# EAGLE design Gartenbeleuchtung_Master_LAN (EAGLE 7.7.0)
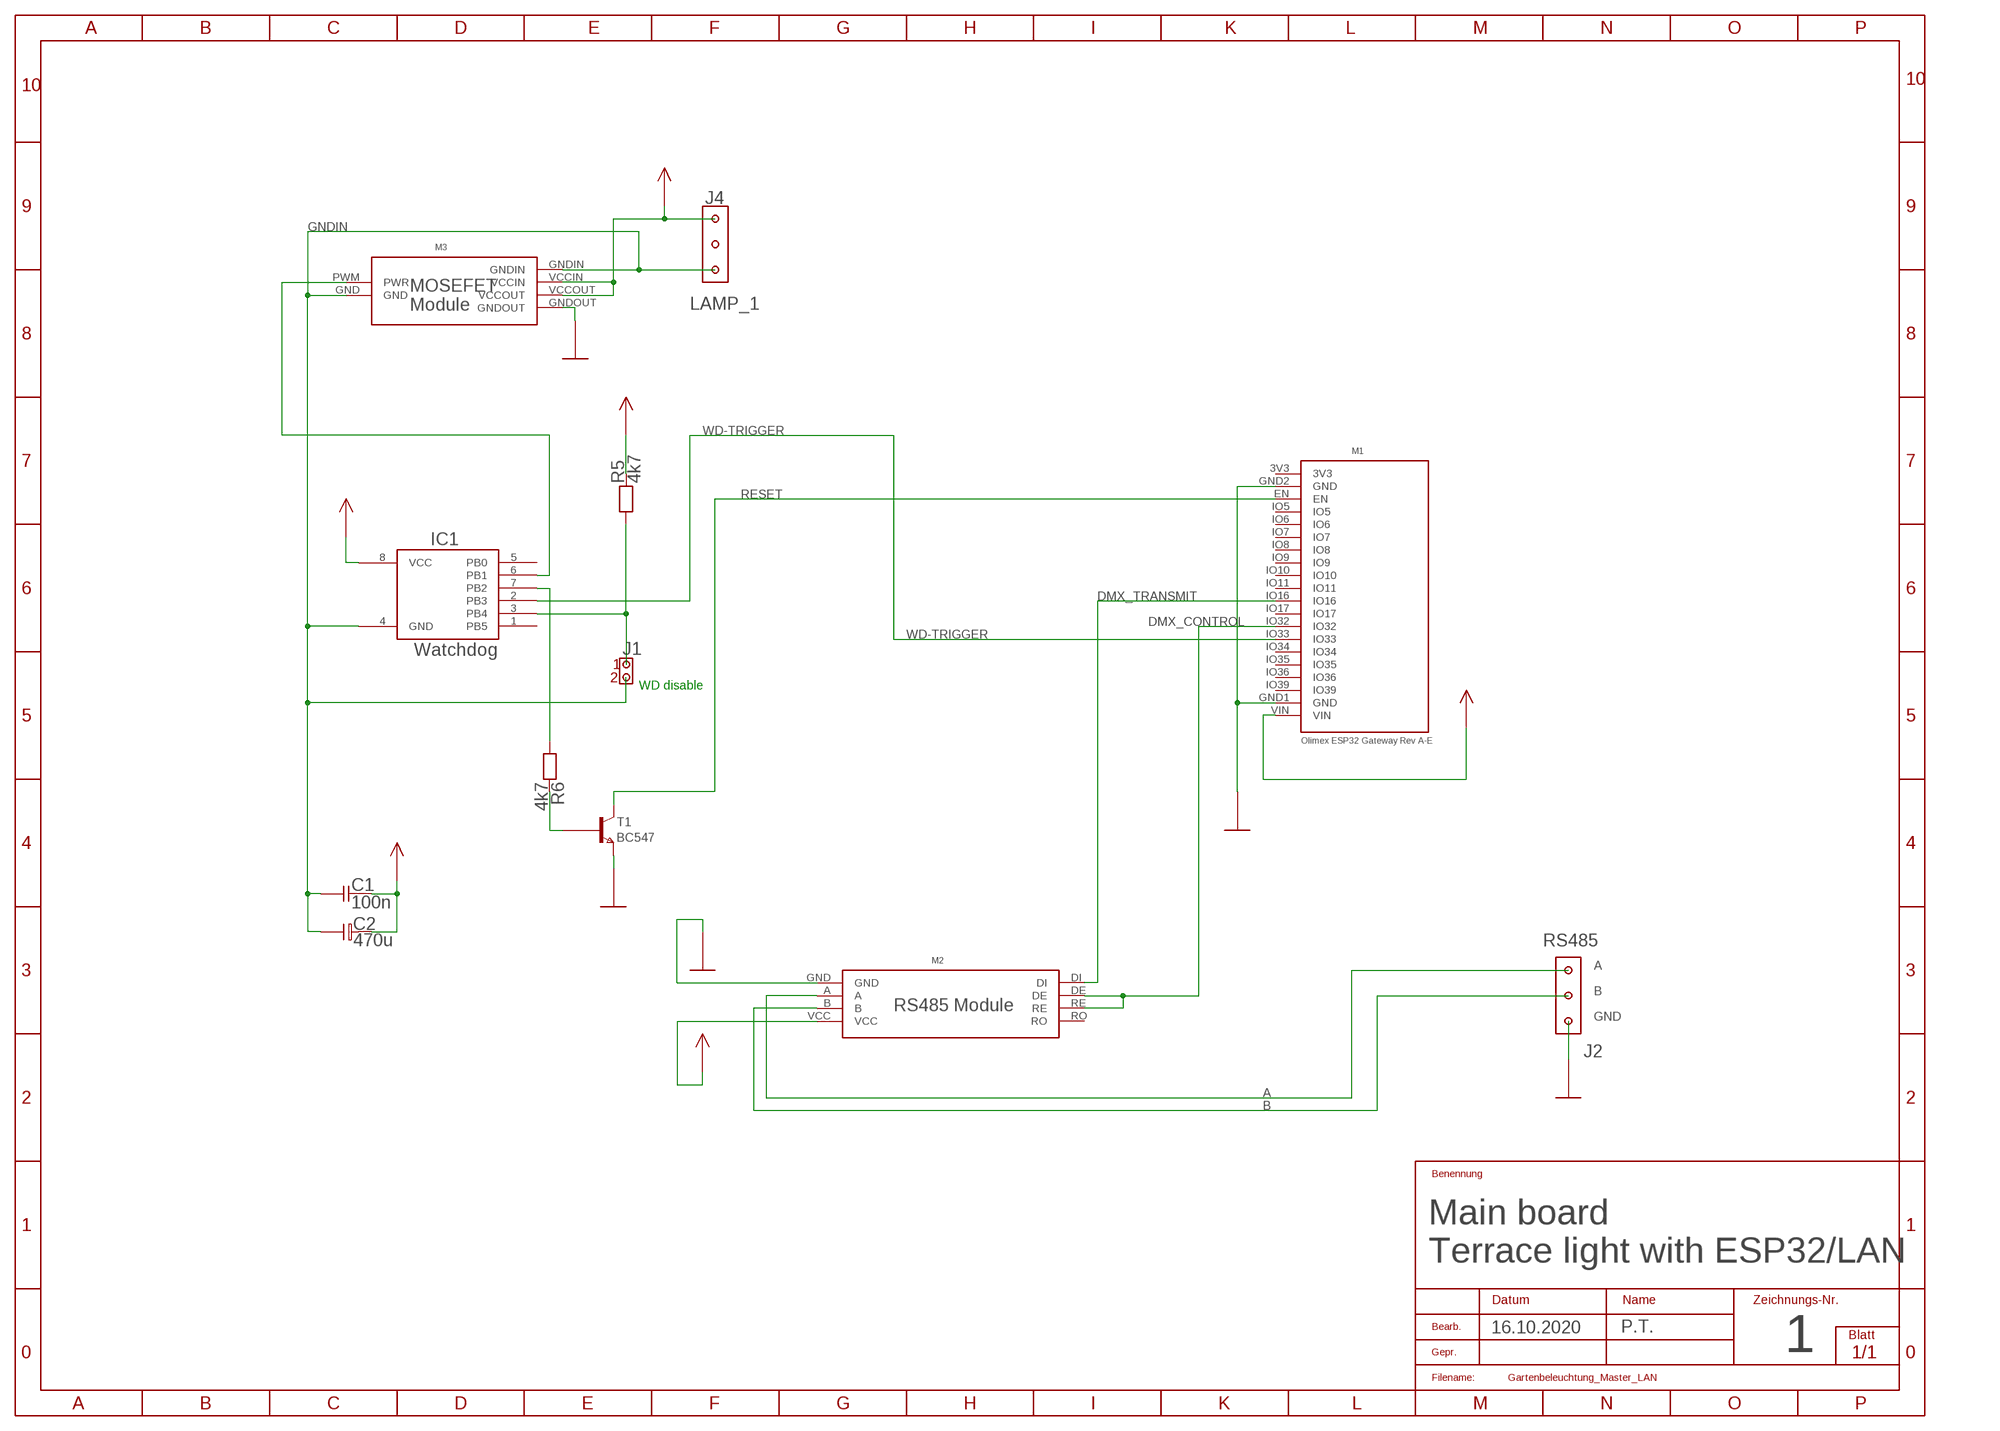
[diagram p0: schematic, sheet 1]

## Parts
C1  100n  CAP02  [CAP02B]
C2  470u  ELK02LI  [ELKOL02B]
IC1  Watchdog  ATINY13A  [DIL8]
J1  WD disable  CON02X1  [CON02X1]
J2  RS485  POWER3X1  [POWER3X1]
J4  LAMP_1  POWER3X1  [POWER3X1]
M1  ESP32-GATEWAY-E  [ESP32-GATEWAY-E]
M2  RS485  [RS485]
M3  MOSFET  [MOSFET]
R5  4k7  RES04  [RES04B]
R6  4k7  RES04  [RES04B]
T1  BC547  BC237  [TO92A]

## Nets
A: J2.3 M2.A
B: J2.2 M2.B
DMX_CONTROL: M1.IO32 M2.DE M2.RE
DMX_TRANSMIT: M1.IO16 M2.DI
GND: J2.1 M1.GND1(GND) M1.GND2(GND) M2.GND M3.GNDOUT T1.3(E)
GNDIN: C1.1 C2.N IC1.4(GND) J1.2 J4.1 M3.GND M3.GNDIN
N$4: IC1.3(PB4) J1.1 R5.1
N$7: IC1.7(PB2) R6.1
N$8: IC1.6(PB1) M3.PWM(PWR)
N$9: R6.2 T1.2(B)
RESET: M1.EN T1.1(C)
VCC: C1.2 C2.P IC1.8(VCC) J4.3 M1.VIN M2.VCC M3.VCCIN M3.VCCOUT R5.2
WD-TRIGGER: IC1.2(PB3) M1.IO33
Unconnected: IC1.1(PB5) IC1.5(PB0) J4.2 M1.IO5 M1.IO6 M1.IO7 M1.IO8 M1.IO9 M1.IO10 M1.IO11 M1.IO17 M1.IO34 M1.IO35 M1.IO36 M1.IO39 M2.RO

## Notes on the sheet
- WD disable
- Main board
- Terrace light with ESP32/LAN
- 16.10.2020 | P.T.
- 1

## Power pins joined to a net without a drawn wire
3V3: M1.3V3

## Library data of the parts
C1 = Discrete:CAP02
C2 = Discrete:ELK02LI
IC1 = Processor:ATINY13A
J1 = Connector 1:CON02X1
J2 J4 = Connector 2:POWER3X1
M1 = Giess:ESP32-GATEWAY-E
M2 = Giess:RS485
M3 = Giess:MOSFET
R5 R6 = Discrete:RES04
T1 = Transistor:BC237

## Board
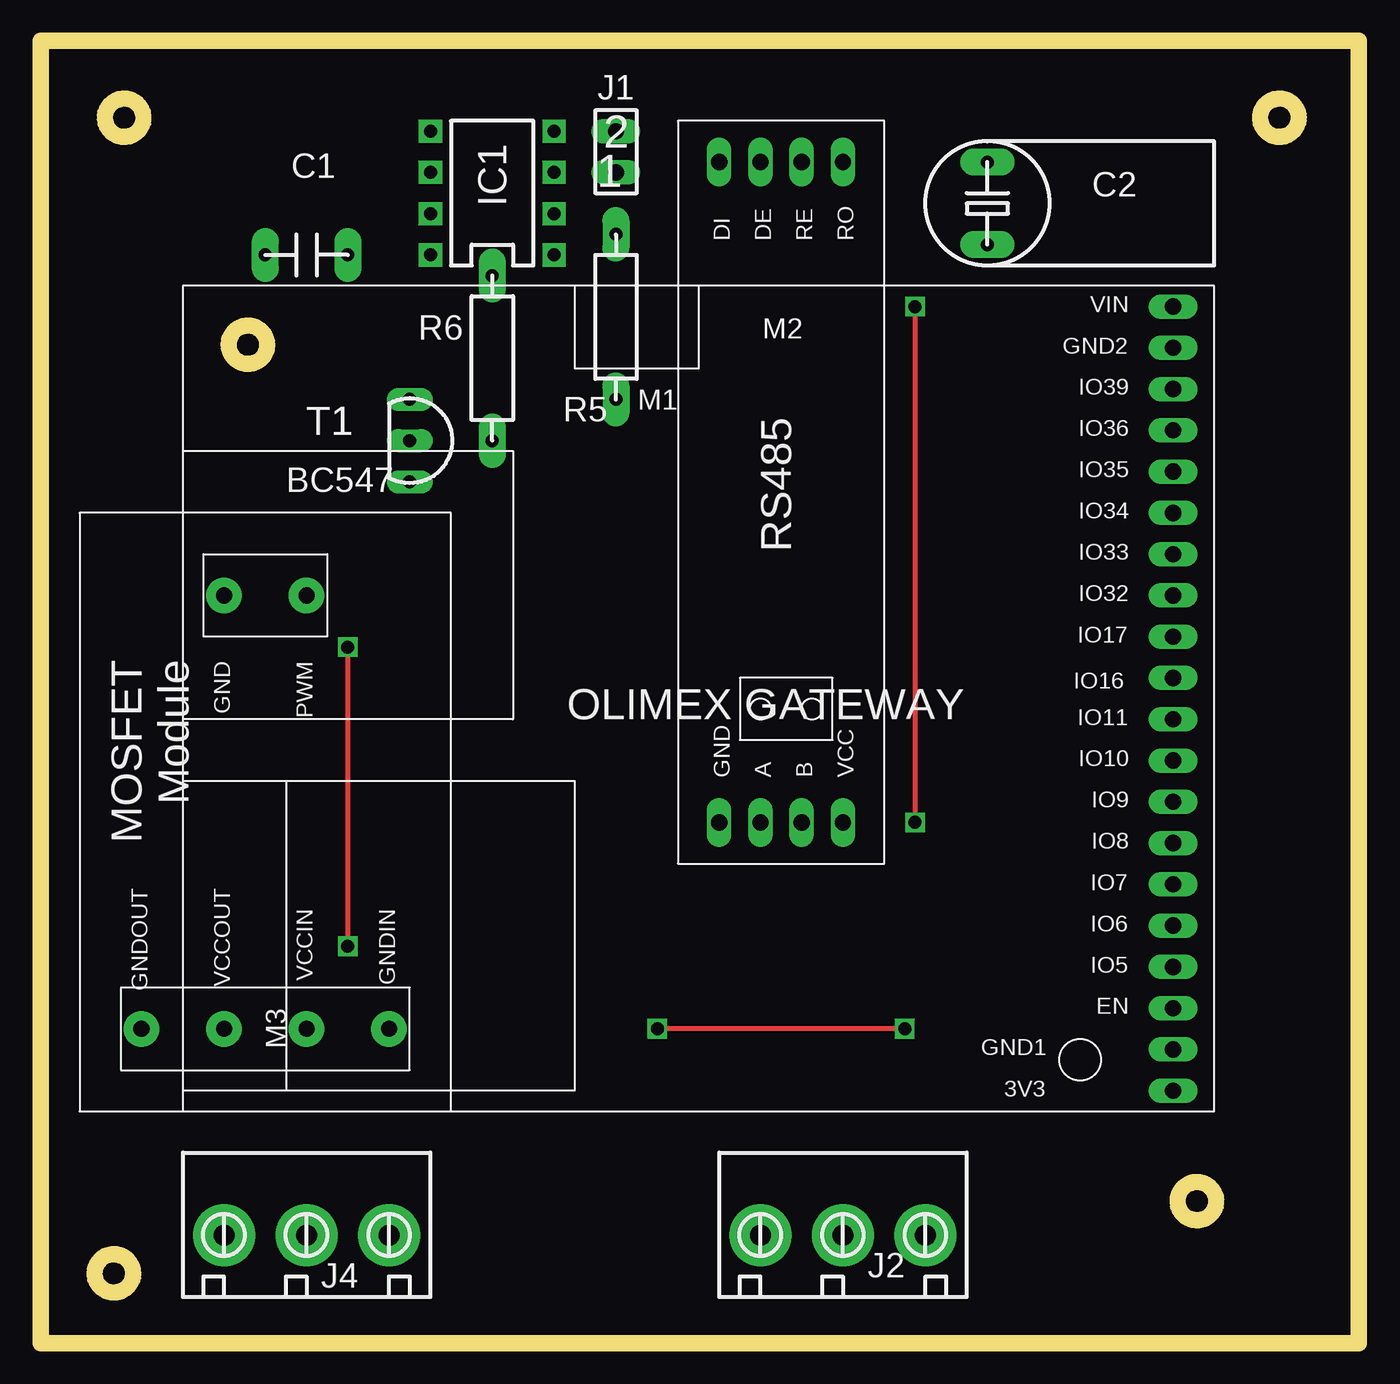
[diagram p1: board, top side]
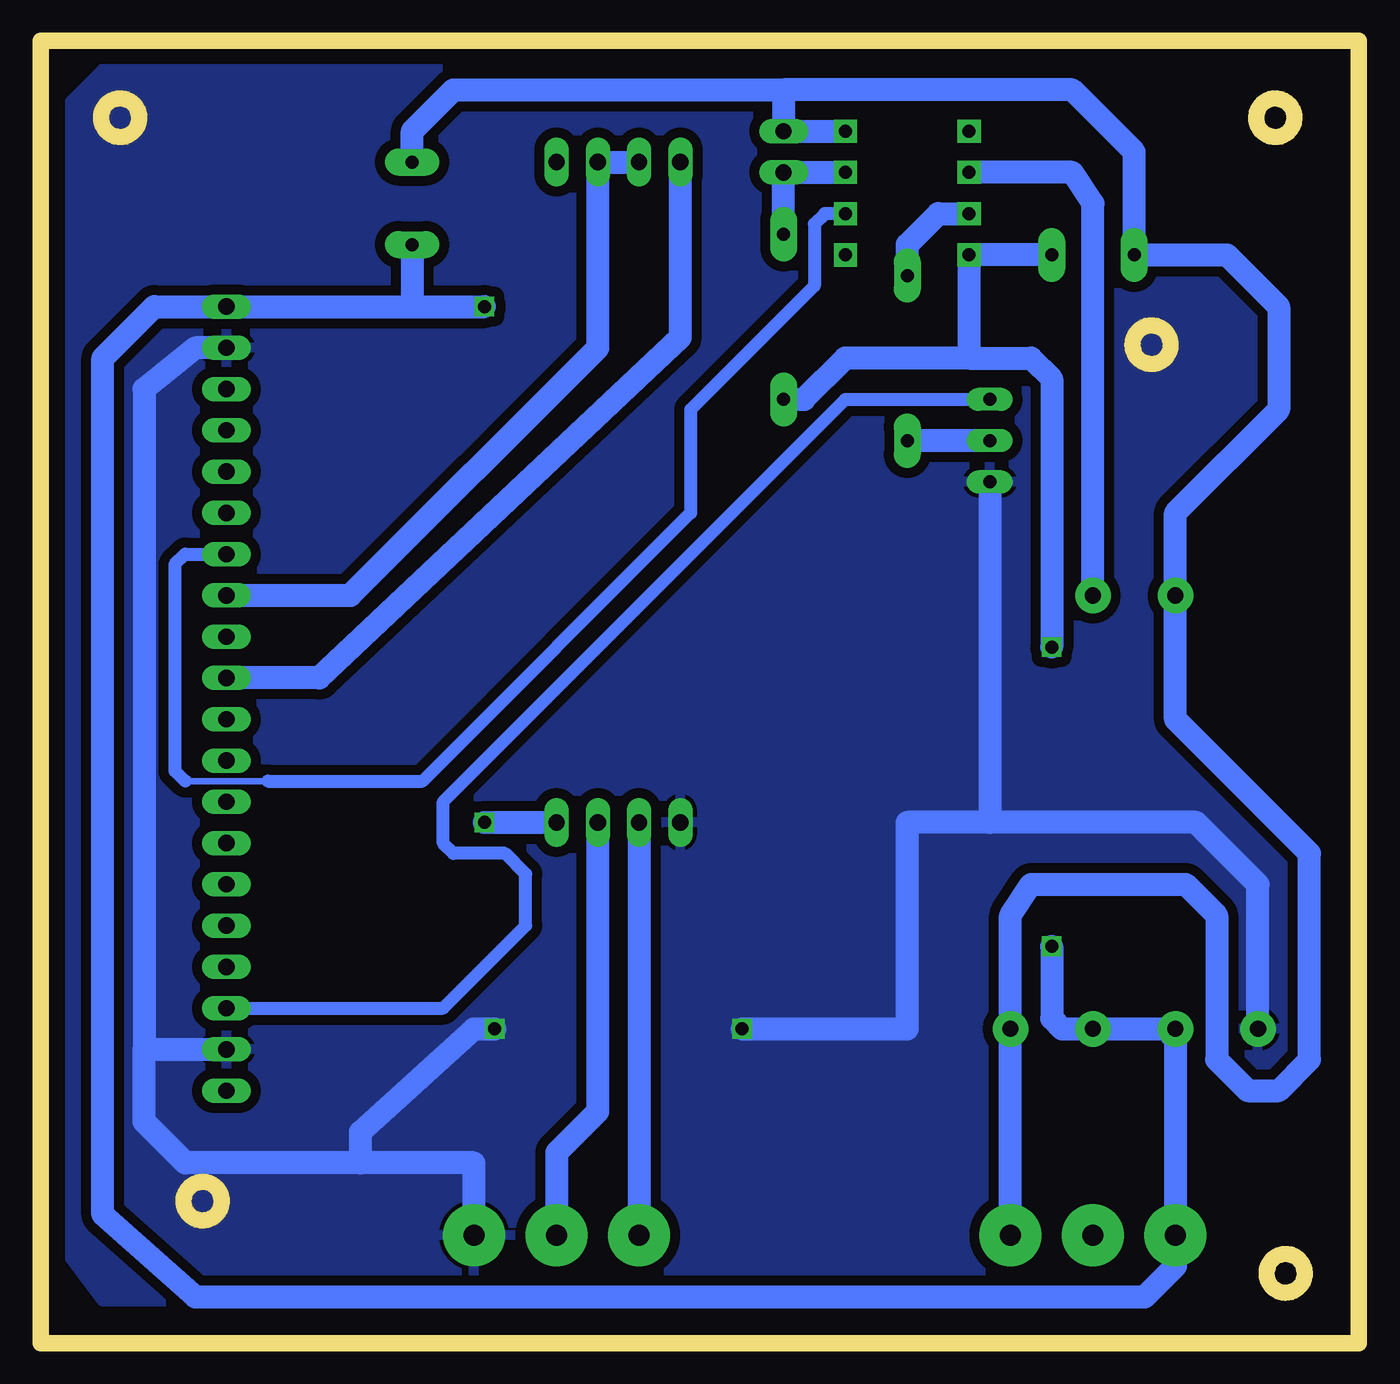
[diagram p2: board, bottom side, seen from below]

Size 81.16 x 80.16 mm. Coordinates in mm from the lower left corner, seen from the top.
Outline: 0,80.16 81.16,80.16 81.16,0 0,0 0,80.16
Copper layers (1*16): Top 0.035mm / dielectric 1.5mm / Bottom 0.035mm
Design rules "default": minimum track width 10mil, minimum drill 24mil, track to track 8mil, track to pad 8mil, pad to pad 8mil, via to via 8mil, smd to smd 8mil, copper to edge 40mil, drill to drill 8mil, minimum pad ring 10mil, minimum via ring 8mil, stop-mask expansion 4mil, vias tented up to drill 0mil, thermal gap 10mil
Milling: 14 lines

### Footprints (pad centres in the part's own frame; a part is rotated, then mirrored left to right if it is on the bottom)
CAP02B = drill 0.8 pad 1.676 long: 1 0,0; 2 5.08,0
ELKOL02B = drill 0.8 pad 1.676 long: N 5.08,0; P 0,0
DIL8 = drill 0.8 pad 1.422 square: 1 0,0; 2 2.54,0; 3 5.08,0; 4 7.62,0; 5 7.62,7.62; 6 5.08,7.62; 7 2.54,7.62; 8 0,7.62
CON02X1 = drill 1 pad 1.422 long: 1 0,0; 2 0,-2.54
POWER3X1 = drill 1.3 pad 3.81: 1 0,0; 2 0,5.08; 3 0,10.16
ESP32-GATEWAY-E = drill 1 pad 1.422 long: 3V3 0,0; EN 0,-5.08; GND1 0,-2.54; GND2 0,-45.72; IO5 0,-7.62; IO6 0,-10.16; IO7 0,-12.7; IO8 0,-15.24; IO9 0,-17.78; IO10 0,-20.32; IO11 0,-22.86; IO16 0,-25.4; IO17 0,-27.94; IO32 0,-30.48; IO33 0,-33.02; IO34 0,-35.56; IO35 0,-38.1; IO36 0,-40.64; IO39 0,-43.18; VIN 0,-48.26
RS485 = drill 1 pad 1.422 long: A -20.32,0; B -20.32,-2.54; DE 20.32,0; DI 20.32,2.54; GND -20.32,2.54; RE 20.32,-2.54; RO 20.32,-5.08; VCC -20.32,-5.08
MOSFET = drill 1 pad 2.184: GND -19.05,-5.08; GNDIN 7.62,5.08; GNDOUT 7.62,-10.16; PWM -19.05,0; VCCIN 7.62,0; VCCOUT 7.62,-5.08
RES04B = drill 0.8 pad 1.676 long: 1 0,0; 2 10.16,0
TO92A = drill 0.8 pad 1.422 long: 1 0,0; 2 2.54,0; 3 5.08,0

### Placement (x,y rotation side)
C1  13.84,66.97 0 top
C2  58.28,67.6 90 top
IC1  31.61,66.97 90 top
J1  35.42,72.05 180 top
J2  54.48,6.64 90 top
J4  21.45,6.64 90 top
M1  69.72,15.53 180 top
M2  44.31,52.36 90 top
M3  16.38,26.96 270 top
R5  35.42,68.23 270 top
R6  27.8,65.69 270 top
T1  22.73,58.07 270 top

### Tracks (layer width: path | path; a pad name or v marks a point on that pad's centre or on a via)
A
  Bottom 1.422: M2.A J2.3
B
  Bottom 1.422: M2.B 46.85,14.26 49.4,11.72 J2.2
DMX_CONTROL
  Bottom 1.422: M1.IO32 62.09,46.01 46.85,61.25 M2.RE M2.DE
DMX_TRANSMIT
  Bottom 1.422: M2.DI 41.77,61.88 64,40.93 M1.IO16
GND  (via drill 0.8 pad 0.81)
  Top 0.305: v53.2,19.34 v37.97,19.34
  Bottom 1.422: J2.1 54.48,11.09 61.46,11.09 | 61.46,11.09 72.25,11.09 74.8,13.62 74.8,18.07 | 74.8,18.07 M1.GND1 | M3.GNDOUT 6.21,28.23 10.03,32.04 22.73,32.04 | 22.73,32.04 27.8,32.04 27.8,19.34 v37.97,19.34 | M1.GND2 71.62,61.25 74.8,58.71 74.8,18.07 | T1.3 22.73,32.04 | 61.46,11.09 61.46,12.99 54.48,19.34 v53.2,19.34
  pour Bottom (isolate 0.61): 3.74,78.39 77.4,78.39 79.37,76.43 79.37,5.18 77.4,2.58 3.74,2.58 1.14,5.81 1.14,76.43
GNDIN
  Bottom 1.422: J4.1 M3.GNDIN 21.45,26.32 20.18,28.23 10.66,28.23 8.76,26.32 8.76,17.44 6.85,15.53 4.95,15.53 3.04,17.44 3.04,30.14 11.29,38.39 M3.GND 11.29,51.09 4.95,57.44 4.95,63.79 8.12,66.97 C1.1 13.84,73.31 17.64,77.12 35.42,77.12 | C2.N 58.28,74.58 55.74,77.12 35.42,77.12 | 35.42,77.12 J1.2 IC1.4
N$4
  Bottom 1.422: IC1.3 J1.1 R5.1
N$7
  Bottom 1.422: R6.1 27.8,67.6 25.9,69.5 IC1.7
N$8
  Bottom 1.422: M3.PWM 16.38,70.14 17.64,72.05 IC1.6
N$9
  Bottom 1.422: T1.2 R6.2
RESET
  Bottom 0.813: M1.EN 56.38,20.61 51.3,25.69 51.3,28.87 52.57,30.14 55.74,30.14 56.38,30.77 56.38,33.31 31.61,58.07 T1.1
VCC  (via drill 0.8 pad 0.81)
  Top 0.305: v53.84,63.79 v53.84,32.04 | v18.91,42.83 v18.91,24.42
  Bottom 1.422: M3.VCCIN M3.VCCOUT | M3.VCCIN 11.93,19.34 11.29,18.71 J4.3 11.29,4.74 13.2,2.83 71.62,2.83 77.33,7.91 77.33,60.61 74.16,63.79 M1.VIN 58.28,63.79 | v53.84,32.04 M2.VCC | 58.28,63.79 v53.84,63.79 | C2.P 58.28,63.79 | C1.2 IC1.8 24,60.61 | 24,60.61 31.61,60.61 34.16,58.07 R5.2 | 24,60.61 20.18,60.61 18.91,59.34 v18.91,42.83 | v18.91,24.42 18.91,19.98 18.28,19.34 M3.VCCIN
WD-TRIGGER
  Bottom 0.406: 72.25,34.58 67.17,34.58
  Bottom 0.813: 72.25,34.58 72.89,35.21 72.89,47.91 72.25,48.55 M1.IO33 | 67.17,34.58 57.65,34.58 41.14,51.09 41.14,57.44 33.52,65.06 33.52,68.87 32.88,69.5 IC1.2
